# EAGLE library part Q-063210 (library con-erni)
Male Connector SMC-Q 50 contacts Standard Assembly Height Source: http://www.erni.com/DB/PDF-Drawing/SMC/063210.pdf
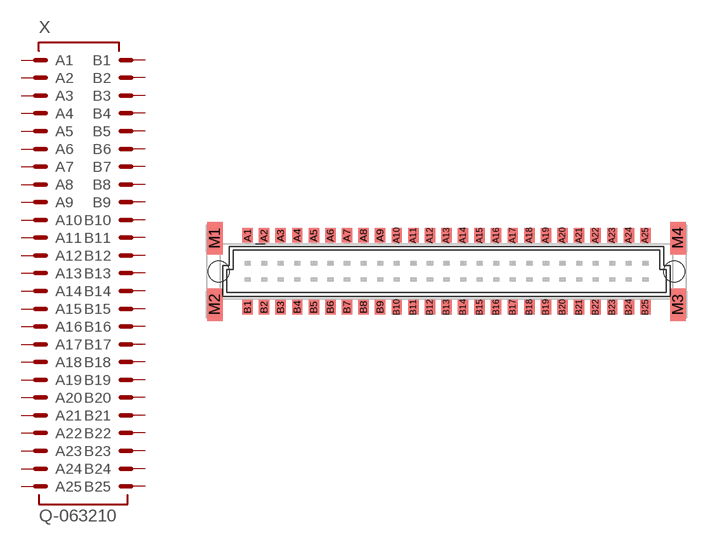
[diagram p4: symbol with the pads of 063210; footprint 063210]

Designator prefix X

## Q-063210 (OC_FARNELL: unknown; OC_NEWARK: unknown)  [063210]
A1  A1  pas
A2  A2  pas
A3  A3  pas
A4  A4  pas
A5  A5  pas
A6  A6  pas
A7  A7  pas
A8  A8  pas
A9  A9  pas
A10  A10  pas
A11  A11  pas
A12  A12  pas
A13  A13  pas
A14  A14  pas
A15  A15  pas
A16  A16  pas
A17  A17  pas
A18  A18  pas
A19  A19  pas
A20  A20  pas
A21  A21  pas
A22  A22  pas
A23  A23  pas
A24  A24  pas
A25  A25  pas
B1  B1  pas
B2  B2  pas
B3  B3  pas
B4  B4  pas
B5  B5  pas
B6  B6  pas
B7  B7  pas
B8  B8  pas
B9  B9  pas
B10  B10  pas
B11  B11  pas
B12  B12  pas
B13  B13  pas
B14  B14  pas
B15  B15  pas
B16  B16  pas
B17  B17  pas
B18  B18  pas
B19  B19  pas
B20  B20  pas
B21  B21  pas
B22  B22  pas
B23  B23  pas
B24  B24  pas
B25  B25  pas

## Footprint 063210 (pad centres in mm)
Male Connector SMC-Q 50 contacts Standard Assembly Height Source: http://www.erni.com/DB/PDF-Drawing/SMC/063210.pdf
smd 0.8 x 1.1: A1 -15.24,2.765; A2 -13.97,2.765; A3 -12.7,2.765; A4 -11.43,2.765; A5 -10.16,2.765; A6 -8.89,2.765; A7 -7.62,2.765; A8 -6.35,2.765; A9 -5.08,2.765; A10 -3.81,2.765; A11 -2.54,2.765; A12 -1.27,2.765; A13 0,2.765; A14 1.27,2.765; A15 2.54,2.765; A16 3.81,2.765; A17 5.08,2.765; A18 6.35,2.765; A19 7.62,2.765; A20 8.89,2.765; A21 10.16,2.765; A22 11.43,2.765; A23 12.7,2.765; A24 13.97,2.765; A25 15.24,2.765; B1 -15.24,-2.74; B2 -13.97,-2.74; B3 -12.7,-2.74; B4 -11.43,-2.74; B5 -10.16,-2.74; B6 -8.89,-2.74; B7 -7.62,-2.74; B8 -6.35,-2.74; B9 -5.08,-2.74; B10 -3.81,-2.74; B11 -2.54,-2.74; B12 -1.27,-2.74; B13 0,-2.74; B14 1.27,-2.74; B15 2.54,-2.74; B16 3.81,-2.74; B17 5.08,-2.74; B18 6.35,-2.74; B19 7.62,-2.74; B20 8.89,-2.74; B21 10.16,-2.74; B22 11.43,-2.74; B23 12.7,-2.74; B24 13.97,-2.74; B25 15.24,-2.74
smd 1.2 x 2.5: M1 -17.745,2.55; M2 -17.745,-2.55; M3 17.745,-2.55; M4 17.745,2.55
hole 1.6 at -17.45,0
hole 1.6 at 17.45,0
